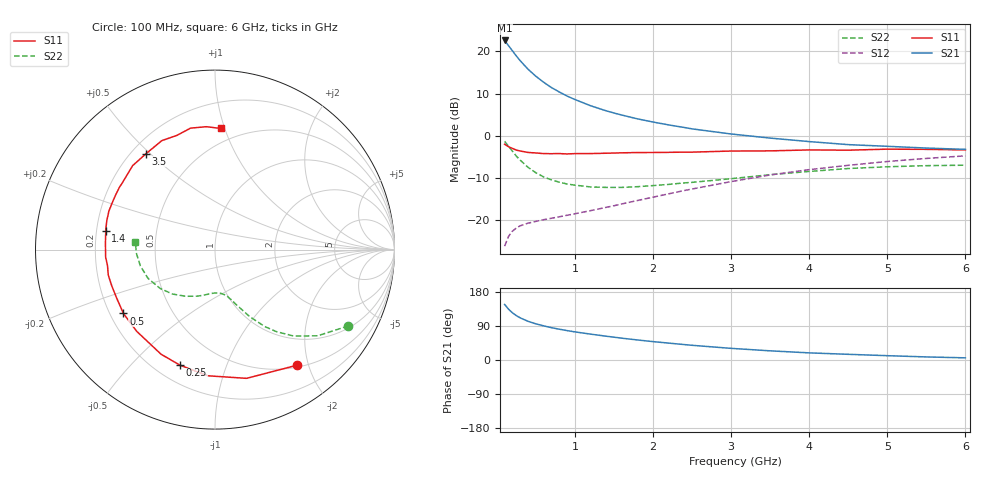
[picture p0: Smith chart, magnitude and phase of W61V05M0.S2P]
! SIEMENS Small Signal Semiconductors
! BFR193W
! Si NPN RF Bipolar Junction Transistor in SOT323
! VCE = 1 V  IC = 5 mA
! Common Emitter S-Parameters:  September  1992
# GHz  S  MA  R  50
!  f  S11  S21  S12  S22
! GHz  MAG  ANG  MAG  ANG  MAG  ANG  MAG  ANG
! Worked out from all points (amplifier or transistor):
!   28 points, 100 MHz to 6 GHz, reference 50 ohm
!   highest |S21| = 22.6 dB at 100 MHz (marker M1)
!   |S21| within 3 dB of that: start of sweep to 222 MHz
!   unconditionally stable (mu >= 1): 1.159 GHz to 2.784 GHz
!   at 300 MHz: K = 0.37, MSG = 19.6 dB, |S12| = -21.4 dB
!   at 1.5 GHz: K = 1.07, MAG = 9.4 dB, |S12| = -16.7 dB
!   at 6 GHz: K = 0.96, MSG = 0.8 dB, |S12| = -4.8 dB
!   S11 on the Smith chart (normalised r, x): 100 MHz: 0.53, -1.81; 250 MHz: 0.30, -0.70; 500 MHz: 0.25, -0.30; 1.4 GHz: 0.24, +0.08; 3.5 GHz: 0.26, +0.49; 6 GHz: 0.39, +0.97
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0.1  0.7893 -54.7  13.52 146.6  0.0485 62.9  0.8561 -29.8
0.15  0.7386 -76.2  11.73 134.1  0.0634 54.0  0.747 -40.0
0.2  0.7042 -93.2  10.18 124.5  0.0731 47.7  0.6527 -47.6
0.25  0.673 -106.8  8.841 117.1  0.0798 43.7  0.5708 -53.2
0.3  0.6558 -117.3  7.759 111.2  0.0847 40.9  0.5105 -57.1
0.4  0.6306 -133.8  6.151 102.1  0.091 38.2  0.4197 -62.7
0.5  0.6219 -145.1  5.072 95.5  0.0956 37.7  0.3618 -66.2
0.6  0.6108 -154.0  4.306 90.1  0.1001 38.1  0.3228 -69.4
0.7  0.6096 -160.7  3.723 85.3  0.1041 39.2  0.2974 -71.6
0.8  0.6114 -166.6  3.299 81.3  0.1084 40.6  0.2794 -73.9
0.9  0.6054 -171.6  2.951 77.6  0.113 42.3  0.2659 -75.6
1  0.6107 -175.9  2.686 74.2  0.1177 43.9  0.2576 -77.8
1.2  0.6115 176.7  2.266 68.3  0.1282 47.1  0.2453 -82.5
1.4  0.6173 170.4  1.97 62.8  0.1403 49.9  0.2422 -86.9
1.8  0.6289 160.1  1.582 52.9  0.1691 54.5  0.247 -96.1
2.2  0.6323 150.6  1.34 44.6  0.2031 57.0  0.263 -104.7
2.5  0.6361 144.4  1.202 38.8  0.2318 57.6  0.2781 -111.1
3  0.6553 134.4  1.045 30.7  0.2839 56.7  0.3074 -122.2
3.5  0.6583 125.6  0.934 24.2  0.3406 53.8  0.3432 -133.9
4.5  0.6707 108.5  0.781 15.0  0.4433 45.3  0.4061 -156.7
5.5  0.6863 94.0  0.711 8.1  0.5353 35.3  0.4392 -177.7
6  0.6759 87.4  0.686 5.7  0.5746 29.9  0.4449 174.7
